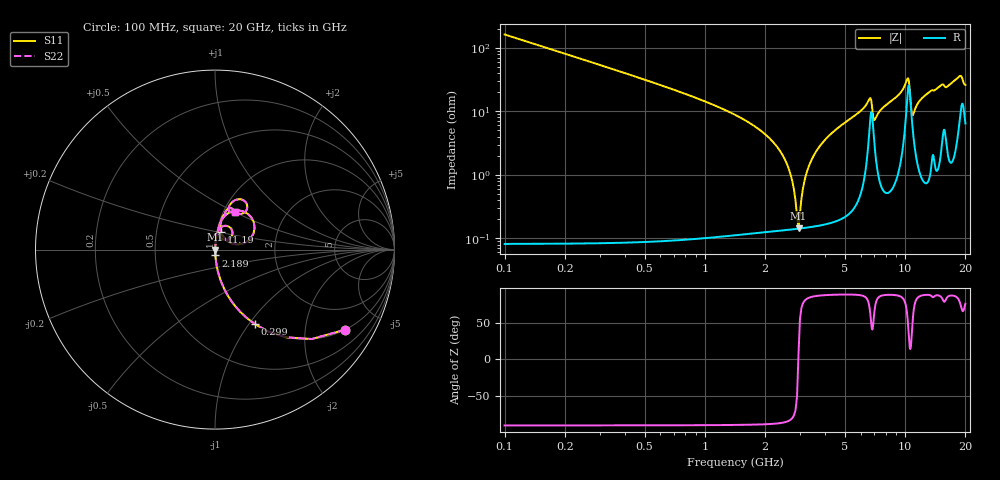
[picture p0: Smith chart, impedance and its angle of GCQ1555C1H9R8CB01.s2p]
!Murata Part Number: GCQ1555C1H9R8CB01
!These Parameters are Measured in Series Mode Connection
!Data Generated on Mar 13, 2026
!  o--ll--o
!Port1  Port2
!  o------o
!Operation Temp=25[degC], DC Bias Voltage=0[V]
!Freq. Start=100[MHz] Stop=20[GHz] 401[Steps]
# Hz S RI R 50
!Freq.(Hz) S11(Real) S11(Imag) S21(Real) S21(Imag) S12(Real) S12(Imag) S22(Real) S22(Imag)
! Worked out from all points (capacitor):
!   401 points, 100 MHz to 20 GHz, reference 50 ohm
!   read as one part in series: C = 9.8 pF near 199.5 MHz
!   lowest |Z| = 143 mohm at 2.936 GHz (marker M1)
!   series resonance near 2.931 GHz, so ESL is about 300 pH
!   S11 on the Smith chart (normalised r, x): 100 MHz: 1.00, -3.24; 299 MHz: 1.00, -1.07; 2.189 GHz: 1.00, -0.07; 11.19 GHz: 1.05, +0.21; 20 GHz: 1.13, +0.51
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1e8  0.7245 -0.4465  0.2755 0.4465  0.2755 0.4465  0.7245 -0.4465
2.99e8  0.2245 -0.4165  0.7755 0.4165  0.7755 0.4165  0.2245 -0.4165
7.4675e8  0.0405 -0.1949  0.9595 0.1949  0.9595 0.1949  0.0405 -0.1949
2.1895e9  0.00237 -0.0328  0.9976 0.0328  0.9976 0.0328  0.00237 -0.0328
2.5875e9  0.00155 -0.0139  0.9984 0.0139  0.9984 0.0139  0.00155 -0.0139
2.73675e9  0.00144 -0.00766  0.9986 0.00766  0.9986 0.00766  0.00144 -0.00766
2.83625e9  0.00142 -0.00367  0.9986 0.00367  0.9986 0.00367  0.00142 -0.00367
2.93575e9  0.00142 0.000189  0.9986 -0.000189  0.9986 -0.000189  0.00142 0.000189
3.1845e9  0.00155 0.00933  0.9984 -0.00933  0.9984 -0.00933  0.00155 0.00933
3.43325e9  0.00184 0.0179  0.9982 -0.0179  0.9982 -0.0179  0.00184 0.0179
4.478e9  0.00437 0.0503  0.9956 -0.0503  0.9956 -0.0503  0.00437 0.0503
6.61725e9  0.0618 0.1327  0.9382 -0.1327  0.9382 -0.1327  0.0618 0.1327
6.7665e9  0.0986 0.0954  0.9014 -0.0954  0.9014 -0.0954  0.0986 0.0954
7.065e9  0.0293 0.0665  0.9707 -0.0665  0.9707 -0.0665  0.0293 0.0665
1.005e10  0.1186 0.2178  0.8814 -0.2178  0.8814 -0.2178  0.1186 0.2178
1.039825e10  0.2207 0.1212  0.7793 -0.1212  0.7793 -0.1212  0.2207 0.1212
1.0846e10  0.0638 0.0521  0.9362 -0.0521  0.9362 -0.0521  0.0638 0.0521
1.119425e10  0.0347 0.0974  0.9653 -0.0974  0.9653 -0.0974  0.0347 0.0974
1.338325e10  0.0507 0.1948  0.9493 -0.1948  0.9493 -0.1948  0.0507 0.1948
1.67165e10  0.078 0.2395  0.922 -0.2395  0.922 -0.2395  0.078 0.2395
1.875625e10  0.16 0.274  0.84 -0.274  0.84 -0.274  0.16 0.274
2e10  0.1106 0.2111  0.8894 -0.2111  0.8894 -0.2111  0.1106 0.2111
